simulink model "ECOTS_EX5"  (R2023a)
settings: Solver=ode23tb  StartTime=0.0  StopTime=1e3  RelTol=1e-3
libraries: component_lib x19, slpidlib x1

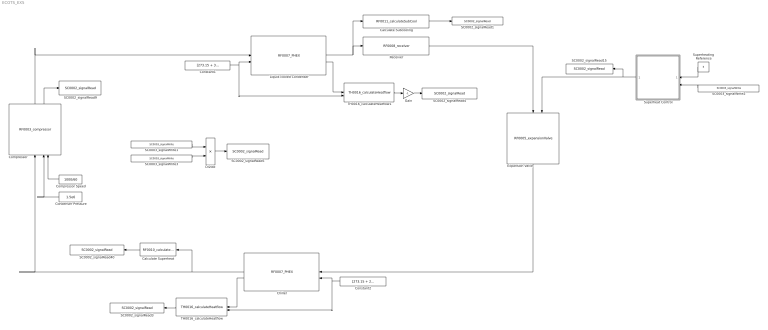
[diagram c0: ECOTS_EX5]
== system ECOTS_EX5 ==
  Calculate Subcooling : component_lib/Thermal Systems/RF0011_calculateSubCool
  Calculate Superheat : component_lib/Thermal Systems/RF0010_calculateSuperHeat
  Chiller : component_lib/Thermal Systems/RF0007_PHEX  N_ch=10  L=180e-3  B=65e-3  H=2e-3  t=0.3e-3  D_h=2.61e-3  N_nod=20
  Compressor : component_lib/Thermal Systems/RF0003_compressor  V_disp=0.00017  N_ref=2000
  Compressor Speed : Constant  Value=1000/60
  Condenser Pressure : Constant  Value=1.5e6
  Constant1 : Constant  Value=[273.15 + 30; 1e5; 0.1]
  Constant2 : Constant  Value=[273.15 + 20; 1e5; 0.05]
  Divide : Product  Inputs=*/
  Expansion Valve : component_lib/Thermal Systems/RF0005_expansionValve  D=3.5*1.8e-3  p_min=100e3
  Gain : Gain  Gain=-1
  Liquid-cooled Condenser : component_lib/Thermal Systems/RF0007_PHEX  N_ch=20  L=180e-3  B=65e-3  H=2e-3  t=0.3e-3  D_h=2.61e-3  N_nod=20
  Receiver : component_lib/Thermal Systems/RF0008_receiver  V=1e-3  h0=280e3  p0=1.6e6  p_gain=1e-2
  SC0002_signalRead1 : component_lib/Data & Control/SC0002_signalRead  SigName=condenserSubCooling
  SC0002_signalRead15 : component_lib/Data & Control/SC0002_signalRead  SigName=expansionValve
  SC0002_signalRead3 : component_lib/Data & Control/SC0002_signalRead  SigName=evaporatorCooling
  SC0002_signalRead4 : component_lib/Data & Control/SC0002_signalRead  SigName=condenserHeating
  SC0002_signalRead40 : component_lib/Data & Control/SC0002_signalRead  SigName=evaporatorSuperheat
  SC0002_signalRead5 : component_lib/Data & Control/SC0002_signalRead  SigName=COOP
  SC0002_signalRead9 : component_lib/Data & Control/SC0002_signalRead  SigName=compressorPower
  SC0003_signalWrite1 : component_lib/Data & Control/SC0003_signalWrite  SigName=evaporatorCooling
  SC0003_signalWrite2 : component_lib/Data & Control/SC0003_signalWrite  SigName=evaporatorSuperheat
  SC0003_signalWrite3 : component_lib/Data & Control/SC0003_signalWrite  SigName=compressorPower
  Superheat Control : Subsystem
  Superheating Reference : Constant  Value=5
  TH0016_calculateHeatflow : component_lib/Thermal Systems/TH0016_calculateHeatflow
  TH0016_calculateHeatflow1 : component_lib/Thermal Systems/TH0016_calculateHeatflow
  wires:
  Calculate Superheat/1 -> SC0002_signalRead40/1
  Compressor Speed/1 -> Compressor/3
  Compressor/1 -> Liquid-cooled Condenser/1
  Compressor/2 -> SC0002_signalRead9/1
  Liquid-cooled Condenser/1 -> Calculate Subcooling/1, Receiver/1
  Receiver/1 -> Expansion Valve/1
  Superheat Control/1(EXV [-]) -> Expansion Valve/2, SC0002_signalRead15/1
  Constant1/1 -> TH0016_calculateHeatflow1/2, Liquid-cooled Condenser/2
  Constant2/1 -> TH0016_calculateHeatflow/2, Chiller/2
  Calculate Subcooling/1 -> SC0002_signalRead1/1
  Chiller/2 -> TH0016_calculateHeatflow/1
  Superheating Reference/1 -> Superheat Control/1(T_ref [K])
  SC0003_signalWrite2/1 -> Superheat Control/2(T_sup [K])
  Condenser Pressure/1 -> Compressor/2
  TH0016_calculateHeatflow/1 -> SC0002_signalRead3/1
  TH0016_calculateHeatflow1/1 -> Gain/1
  Gain/1 -> SC0002_signalRead4/1
  Liquid-cooled Condenser/2 -> TH0016_calculateHeatflow1/1
  SC0003_signalWrite1/1 -> Divide/1
  SC0003_signalWrite3/1 -> Divide/2
  Divide/1 -> SC0002_signalRead5/1
  Chiller/1 -> Compressor/1, Calculate Superheat/1
  Expansion Valve/1 -> Chiller/1

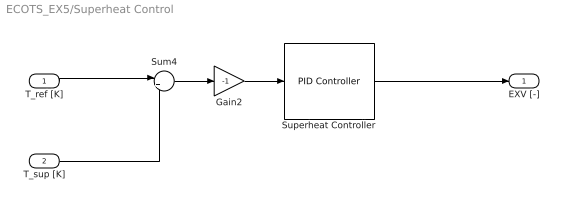
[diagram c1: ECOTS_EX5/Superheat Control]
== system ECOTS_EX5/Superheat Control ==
  T_ref [K] : Inport
  T_sup [K] : Inport  Port=2
  Gain2 : Gain  Gain=-1
  Sum4 : Sum  Inputs=|+-
  Superheat Controller : slpidlib/PID Controller  Controller=PI  Form=Parallel  TimeDomain=Continuous-time  UseExternalTs=off  SampleTime=-1  IntegratorMethod=Forward Euler  FilterMethod=Forward Euler  ControllerParametersSource=internal  P=1e-2  I=1e-2  UseKiTs=off  D=0  N=100  UseFilter=on  TunerSelectOption=Transfer Function Based (PID Tuner App)  InitialConditionSource=internal  InitialConditionForIntegrator=0.3  InitialConditionForFilter=0  DifferentiatorICPrevScaledInput=0  ExternalReset=none  TrackingMode=off  Kt=1  LimitOutput=on  SatLimitsSource=internal  UpperSaturationLimit=1  LowerSaturationLimit=0  LinearizeAsGain=on  AntiWindupMode=clamping  Kb=1  LimitIntegrator=off  UpperIntegratorSaturationLimit=inf  LowerIntegratorSaturationLimit=-inf  POutMin=[]  POutMax=[]  IOutMin=[]  IOutMax=[]  DOutMin=[]  DOutMax=[]  NOutMin=[]  NOutMax=[]  SumOutMin=[]  SumOutMax=[]  SaturationOutMin=[]  SaturationOutMax=[]  PParamMin=[]  PParamMax=[]  IParamMin=[]  IParamMax=[]  DParamMin=[]  DParamMax=[]  NParamMin=[]  NParamMax=[]  KbParamMin=[]  KbParamMax=[]  KtParamMin=[]  KtParamMax=[]  KbOutMin=[]  KbOutMax=[]  KtOutMin=[]  KtOutMax=[]  IntegratorOutMin=[]  IntegratorOutMax=[]  FilterOutMin=[]  FilterOutMax=[]  SumI1OutMin=[]  SumI1OutMax=[]  SumI2OutMin=[]  SumI2OutMax=[]  SumI3OutMin=[]  SumI3OutMax=[]  SumI4OutMin=[]  SumI4OutMax=[]  SumDOutMin=[]  SumDOutMax=[]  DifferentiatorOutMin=[]  DifferentiatorOutMax=[]  FilterDiffOutCoefMin=[]  FilterDiffOutCoefMax=[]  ReciprocalOutMin=[]  ReciprocalOutMax=[]  SumDenOutMin=[]  SumDenOutMax=[]  SumNumOutMin=[]  SumNumOutMax=[]  DivideOutMin=[]  DivideOutMax=[]  UdiffTsProdOutMin=[]  UdiffTsProdOutMax=[]  NTsProdOutMin=[]  NTsProdOutMax=[]  UintegralTsProdOutMin=[]  UintegralTsProdOutMax=[]  UngainTsProdOutMin=[]  UngainTsProdOutMax=[]  ClampingZeroOutDataTypeStr=Inherit: Inherit via back propagation  ClampingZeroOutMin=[]  ClampingZeroOutMax=[]  FilterDenConstantOutDataTypeStr=Inherit: Inherit via back propagation  FilterDenConstantOutMin=[]  FilterDenConstantOutMax=[]  PCopyOutDataTypeStr=Inherit: Inherit via back propagation  PCopyOutMin=[]  PCopyOutMax=[]  NCopyOutDataTypeStr=Inherit: Inherit via back propagation  NCopyOutMin=[]  NCopyOutMax=[]  IntegratorContinuousStateAttributes=''  IntegratorStateMustResolveToSignalObject=off  IntegratorRTWStateStorageClass=Auto  FilterContinuousStateAttributes=''  FilterStateMustResolveToSignalObject=off  FilterRTWStateStorageClass=Auto  ParallelPVariant=InternalParameters  IdealPVariant=Disabled  IVariant=InternalParameters  DVariant=Disabled  IntegratorVariant=Continuous  SatVariant=Enabled  AWVariant=ContClampingParallel  PCopyVariant=Disabled  TRVariant=Disabled  FdbkBlocksVariant=Forward  IdealPFdbkVariant=Disabled  SatFdbkVariant=Disabled  DerivativeFilterVariant=Disabled  NVariant=Disabled  NCopyVariant=Disabled_SignalSpec  FilterICVariant=Disabled  IntegratorICVariant=InternalICs  ExternalResetVariant=Disabled  TRSumVariant=Passthrough  SumFdbkVariant=Disabled  SumVariant=Sum_PI  TsampFilterVariant=InternalTs  TsampNgainVariant=Passthrough  TsampIntegralVariant=Disabled_SignalSpec  ExternalSaturationOutDataTypeStr=Inherit: Same as second input
  EXV [-] : Outport
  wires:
  Sum4/1 -> Gain2/1
  T_ref [K]/1 -> Sum4/1
  T_sup [K]/1 -> Sum4/2
  Gain2/1 -> Superheat Controller/1
  Superheat Controller/1 -> EXV [-]/1
